(* Logix 5000 DataType export wxsSystemControl; software revision 32.00 *)

TYPE wxsPushbutton :
STRUCT
   Active : BOOL;   // Mouse Click
   Enable : BOOL;   // Enable/Disable
END_STRUCT
END_TYPE

TYPE wxsSystemControl :   // Revolution St. WXS UDT
STRUCT
   SystemStart : wxsPushbutton;   // Global Start
   SystemStop : wxsPushbutton;   // Global Stop
   SystemReset : wxsPushbutton;   // Global Reset
   SystemEmergencyStop : wxsPushbutton;   // Emergency Stop
   SystemStatus : STRING;   // Global System Status
   SystemShiftActive : BOOL;   // Shift Active
END_STRUCT
END_TYPE
